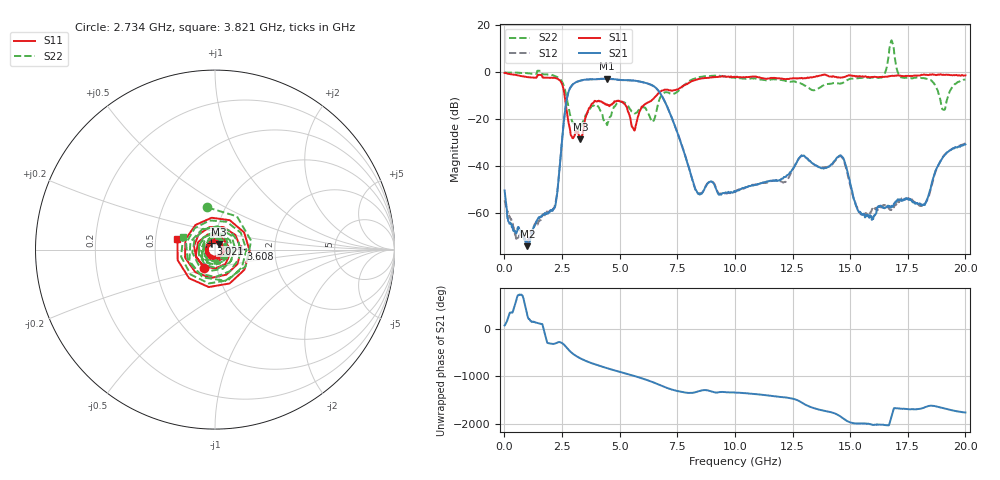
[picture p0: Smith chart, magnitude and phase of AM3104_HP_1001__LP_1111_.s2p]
!Created with skrf (http://scikit-rf.org).
# Hz S RI R 50.0
!freq ReS11 ImS11 ReS21 ImS21 ReS12 ImS12 ReS22 ImS22
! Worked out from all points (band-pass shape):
!   1601 points, 10 MHz to 20 GHz, reference 50 ohm
!   highest |S21| = -2.68 dB at 4.458 GHz (marker M1); lowest = -74.1 dB at 997 MHz (marker M2)
!   |S21| within 3 dB of the highest: 2.919 GHz to 6.445 GHz (3.527 GHz wide, 75.3 % of centre)
!   lowest |S11| = -28.5 dB at 3.296 GHz (marker M3), VSWR 1.08, Z = 52 + j3.27 ohm
!   |S11| at or under -10 dB: 2.614 GHz to 6.585 GHz (3.971 GHz wide, 86.3 % of centre)
!   |S22| runs from -24.6 to 13.6 dB; largest |S21 - S12| = 0.083
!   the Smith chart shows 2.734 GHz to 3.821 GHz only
!   S11 on the Smith chart (normalised r, x): 2.734 GHz: 0.86, -0.18; 3.021 GHz: 0.95, +0.07; 3.608 GHz: 1.34, +0.01; 3.821 GHz: 0.65, +0.08
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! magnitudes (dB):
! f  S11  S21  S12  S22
! 10 MHz  -0.2  -50.3  -54.6  0.0
! 997 MHz  -2.0  -74.1  -72.1  -0.4
! 2.184 GHz  -2.4  -57.7  -57.0  -1.5
! 2.734 GHz  -18.3  -10.2  -10.2  -12.4
! 3.021 GHz  -27.5  -4.8  -4.8  -21.5
! 3.296 GHz  -28.5  -3.5  -3.6  -23.5
! 3.346 GHz  -27.0  -3.4  -3.4  -23.0
! 3.608 GHz  -16.8  -3.0  -3.1  -17.2
! 3.821 GHz  -13.2  -2.9  -2.9  -14.4
! 4.458 GHz  -13.7  -2.7  -2.7  -22.5
! 5.62 GHz  -24.4  -3.5  -3.5  -17.3
! 6.682 GHz  -8.9  -7.8  -7.8  -12.9
! 8.381 GHz  -3.0  -51.3  -51.2  -2.1
! 10.01 GHz  -2.0  -50.7  -50.9  -2.4
! 13.34 GHz  -2.2  -38.6  -38.6  -7.5
! 14.62 GHz  -2.2  -35.6  -36.0  -4.7
! 15.43 GHz  -1.7  -59.4  -59.7  -2.4
! 16.4 GHz  -1.9  -57.6  -56.8  -1.9
! 16.68 GHz  -1.7  -57.2  -58.0  7.3
! 18.2 GHz  -0.9  -56.5  -56.6  -2.5
! 19.05 GHz  -1.0  -35.8  -35.7  -15.9
! 20 GHz  -1.3  -30.7  -30.3  -3.0
